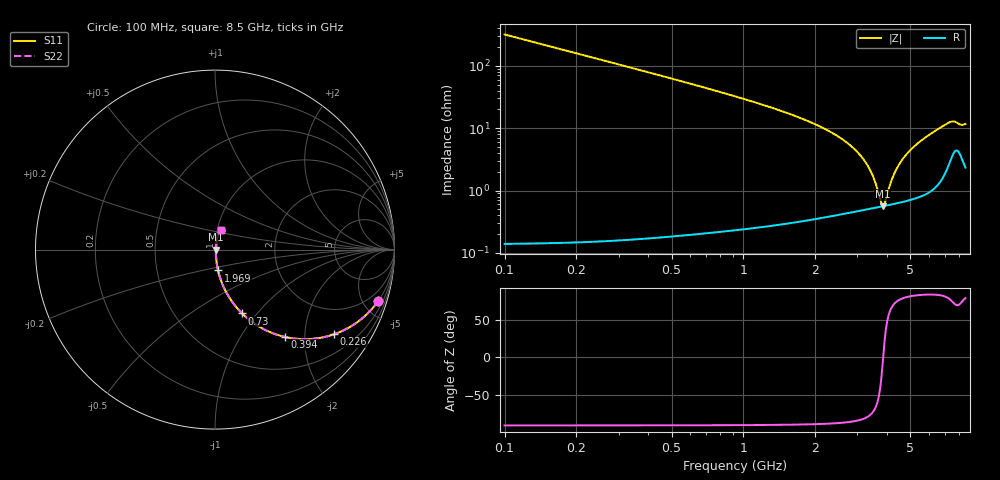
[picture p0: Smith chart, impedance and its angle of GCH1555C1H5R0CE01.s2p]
!Murata Part Number: GCH1555C1H5R0CE01
!These Parameters are Measured in Series Mode Connection
!Data Generated on Jun 19, 2026
!  o--ll--o
!Port1  Port2
!  o------o
!Operation Temp=25[degC], DC Bias Voltage=0[V]
!Freq. Start=100[MHz] Stop=9[GHz] 401[Steps]
# Hz S RI R 50
!Freq.(Hz) S11(Real) S11(Imag) S21(Real) S21(Imag) S12(Real) S12(Imag) S22(Real) S22(Imag)
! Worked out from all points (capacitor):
!   401 points, 100 MHz to 8.5 GHz, reference 50 ohm
!   read as one part in series: C = 5 pF near 142 MHz
!   lowest |Z| = 563 mohm at 3.838 GHz (marker M1)
!   series resonance near 3.847 GHz, so ESL is about 340 pH
!   S11 on the Smith chart (normalised r, x): 100 MHz: 1.00, -6.36; 226 MHz: 1.00, -2.81; 394 MHz: 1.00, -1.60; 730 MHz: 1.00, -0.84; 1.969 GHz: 1.01, -0.24; 8.5 GHz: 1.05, +0.23
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1e8  0.9099 -0.286  0.0901 0.286  0.0901 0.286  0.9099 -0.286
2.26e8  0.663 -0.4721  0.337 0.4721  0.337 0.4721  0.663 -0.4721
3.94e8  0.3898 -0.4866  0.6102 0.4866  0.6102 0.4866  0.3898 -0.4866
5.41e8  0.2499 -0.4313  0.7501 0.4313  0.7501 0.4313  0.2499 -0.4313
7.3e8  0.1509 -0.3555  0.8491 0.3555  0.8491 0.3555  0.1509 -0.3555
1.045e9  0.0753 -0.2595  0.9247 0.2595  0.9247 0.2595  0.0753 -0.2595
1.507e9  0.0334 -0.1716  0.9666 0.1716  0.9666 0.1716  0.0334 -0.1716
1.969e9  0.0172 -0.1161  0.9828 0.1161  0.9828 0.1161  0.0172 -0.1161
2.914e9  0.00664 -0.0457  0.9934 0.0457  0.9934 0.0457  0.00664 -0.0457
3.397e9  0.0055 -0.0202  0.9945 0.0202  0.9945 0.0202  0.0055 -0.0202
3.565e9  0.00543 -0.0124  0.9946 0.0124  0.9946 0.0124  0.00543 -0.0124
3.775e9  0.00552 -0.00306  0.9945 0.00306  0.9945 0.00306  0.00552 -0.00306
3.838e9  0.00558 -0.000368  0.9944 0.000368  0.9944 0.000368  0.00558 -0.000368
3.901e9  0.00566 0.00228  0.9943 -0.00228  0.9943 -0.00228  0.00566 0.00228
4.111e9  0.00601 0.0108  0.994 -0.0108  0.994 -0.0108  0.00601 0.0108
4.3e9  0.00644 0.0182  0.9936 -0.0182  0.9936 -0.0182  0.00644 0.0182
4.531e9  0.00711 0.0268  0.9929 -0.0268  0.9929 -0.0268  0.00711 0.0268
4.846e9  0.00826 0.038  0.9917 -0.038  0.9917 -0.038  0.00826 0.038
5.707e9  0.0129 0.0667  0.9871 -0.0667  0.9871 -0.0667  0.0129 0.0667
7.114e9  0.0339 0.11  0.9661 -0.11  0.9661 -0.11  0.0339 0.11
7.534e9  0.0495 0.1127  0.9505 -0.1127  0.9505 -0.1127  0.0495 0.1127
8.5e9  0.035 0.1079  0.965 -0.1079  0.965 -0.1079  0.035 0.1079
